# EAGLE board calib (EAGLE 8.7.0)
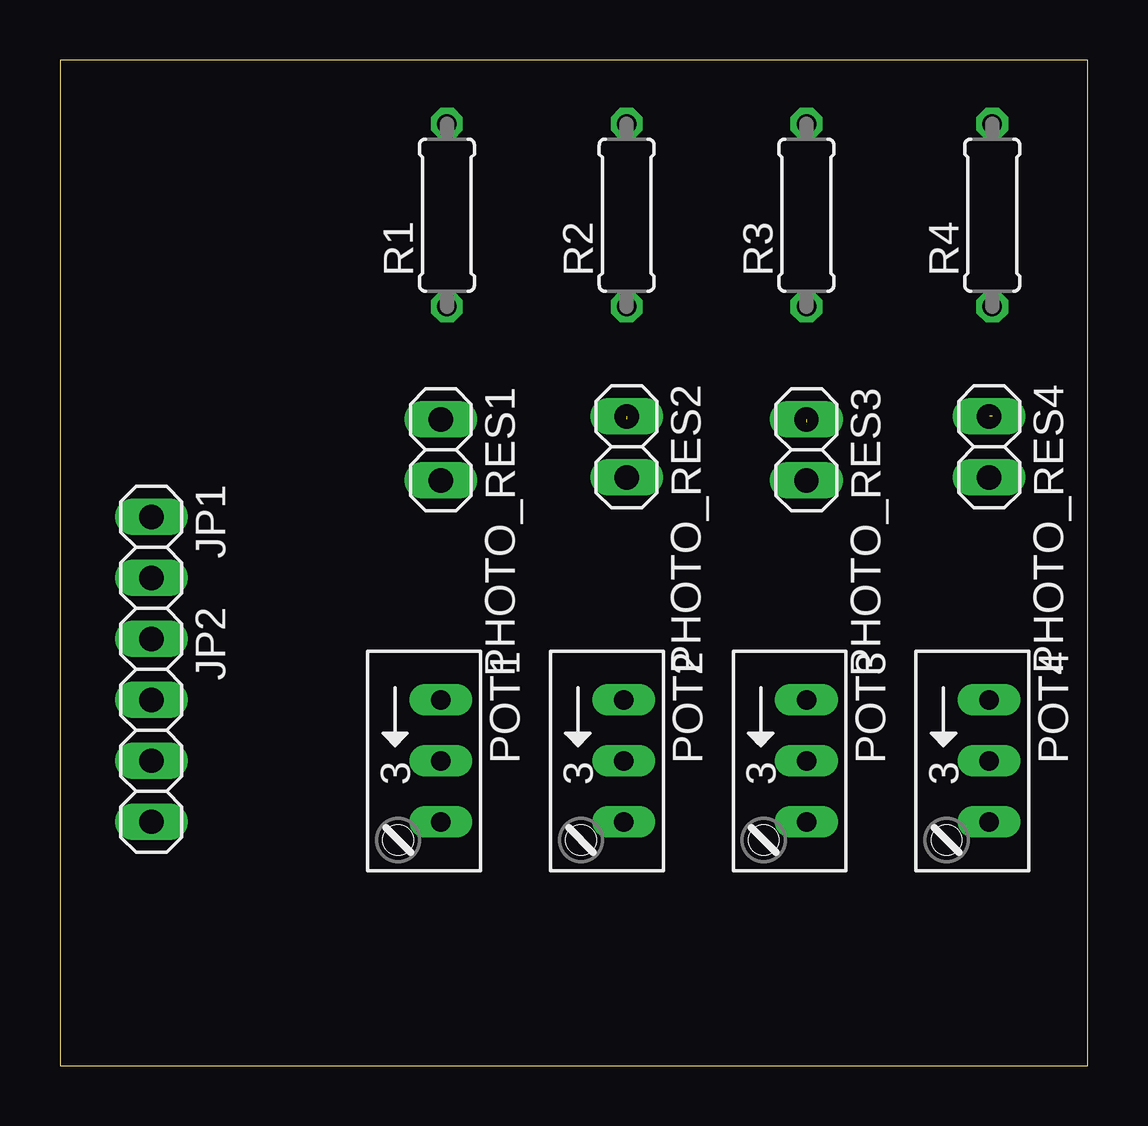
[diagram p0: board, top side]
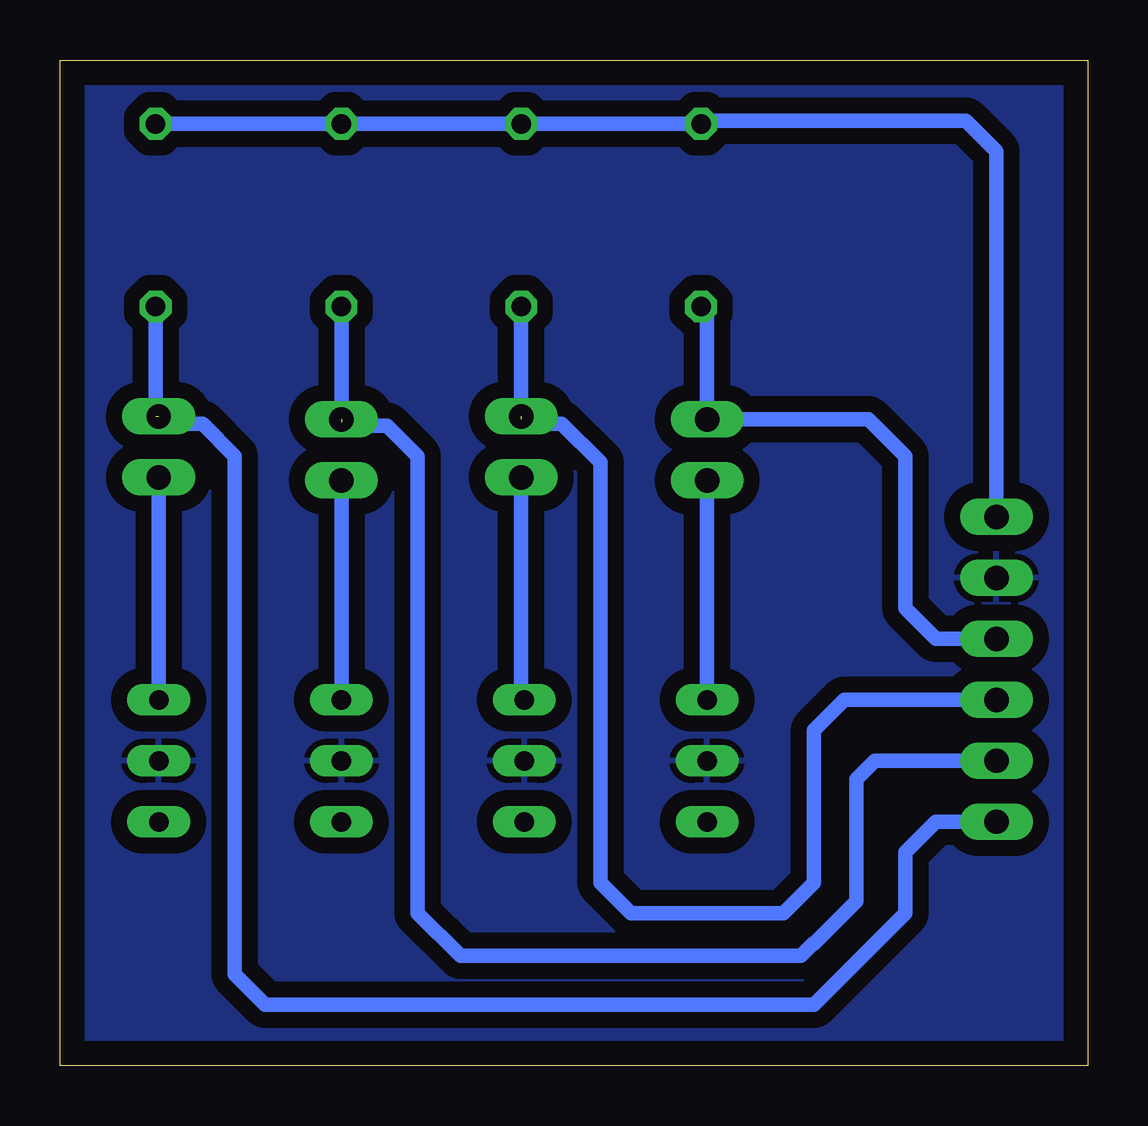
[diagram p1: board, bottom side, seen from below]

Size 42.85 x 41.9 mm. Coordinates in mm from the lower left corner, seen from the top.
Outline: 0,0 42.85,0 42.85,41.9 0,41.9 0,0
Copper layers (1*16): Top 0.035mm / dielectric 1.5mm / Bottom 0.035mm
Design rules "default *": minimum track width 6mil, minimum drill 0.35mm, track to track 26mil, track to pad 26mil, pad to pad 6mil, via to via 6mil, smd to smd 6mil, copper to edge 40mil, drill to drill 6mil, minimum pad ring 10mil, minimum via ring 8mil, stop-mask expansion 4mil, vias tented up to drill 0mil, thermal gap 10mil

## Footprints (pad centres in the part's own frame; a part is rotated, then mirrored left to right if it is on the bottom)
1X02 = drill 1.016 long: 1 -1.27,0; 2 1.27,0
1X04 = drill 1.016 long: 1 -3.81,0; 2 -1.27,0; 3 1.27,0; 4 3.81,0
RJ9W = drill 0.813 long: A 2.54,0.635; E -2.54,0.635; S 0,0.635
0207/7 = drill 0.813 octagon: 1 -3.81,0; 2 3.81,0

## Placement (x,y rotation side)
JP1  [1X02]  3.81,21.59 270 top
JP2  [1X04]  3.81,13.97 270 top
PHOTO_RES1  [1X02]  15.88,25.65 270 top
PHOTO_RES2  [1X02]  23.62,25.78 270 top
PHOTO_RES3  [1X02]  31.11,25.65 270 top
PHOTO_RES4  [1X02]  38.73,25.78 270 top
POT1  [RJ9W]  15.24,12.7 270 top
POT2  [RJ9W]  22.86,12.7 270 top
POT3  [RJ9W]  30.48,12.7 270 top
POT4  [RJ9W]  38.1,12.7 270 top
R1  [0207/7]  16.13,35.43 90 top
R2  [0207/7]  23.62,35.43 90 top
R3  [0207/7]  31.11,35.43 90 top
R4  [0207/7]  38.86,35.43 90 top

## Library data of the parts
JP1 JP2 PHOTO_RES1-PHOTO_RES4 = pinhead
POT1-POT4 = pot
R1-R4 = rcl; SPICEPREFIX: R

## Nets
GND: JP1.2 POT1.S POT2.S POT3.S POT4.S
N$1: JP2.1 PHOTO_RES1.1 R1.1
N$2: PHOTO_RES1.2 POT1.E
N$3: JP2.2 PHOTO_RES2.1 R2.1
N$4: PHOTO_RES2.2 POT2.E
N$5: JP2.3 PHOTO_RES3.1 R3.1
N$6: PHOTO_RES3.2 POT3.E
N$7: JP2.4 PHOTO_RES4.1 R4.1
N$8: PHOTO_RES4.2 POT4.E
VCC: JP1.1 R1.2 R2.2 R3.2 R4.2

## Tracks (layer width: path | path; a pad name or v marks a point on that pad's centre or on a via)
GND
  pour Bottom: -1.27,43.18 -1.27,-1.27 44.45,-1.27 44.45,43.18
N$1
  Bottom 0.61: R1.1 15.88,31.37 PHOTO_RES1.1 9.14,26.92 7.62,25.4 7.62,19.05 6.35,17.78 JP2.1
N$2
  Bottom 0.61: PHOTO_RES1.2 POT1.E
N$3  (1 unrouted)
  Bottom 0.61: R2.1 23.62,26.92 | PHOTO_RES2.1 23.32,26.75 21.93,26.75 20.32,25.13 20.32,7.62 19.05,6.35 12.7,6.35 11.43,7.62 11.43,13.97 10.16,15.24 JP2.2
N$4
  Bottom 0.406: 23.62,15.37 POT2.E
  Bottom 0.61: PHOTO_RES2.2 23.62,15.37
N$5  (1 unrouted)
  Bottom 0.61: R3.1 31.11,26.8 | PHOTO_RES3.1 30.86,26.67 29.21,26.67 27.94,25.4 27.94,6.35 26.16,4.57 11.96,4.57 11.46,5.08 11.43,5.08 9.65,6.86 9.65,11.94 8.89,12.7 JP2.3
N$6
  Bottom 0.61: PHOTO_RES3.2 POT3.E
N$7  (1 unrouted)
  Bottom 0.61: R4.1 38.86,27.05 38.56,26.75 36.91,26.75 35.56,25.4 35.56,3.81 34.29,2.54 11.43,2.54 7.62,6.35 7.62,8.89 6.35,10.16 JP2.4
N$8
  Bottom 0.61: PHOTO_RES4.2 POT4.E
VCC
  Bottom 0.61: JP1.1 3.81,38.1 5.08,39.37 16,39.37 R1.2 R2.2 R3.2 R4.2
